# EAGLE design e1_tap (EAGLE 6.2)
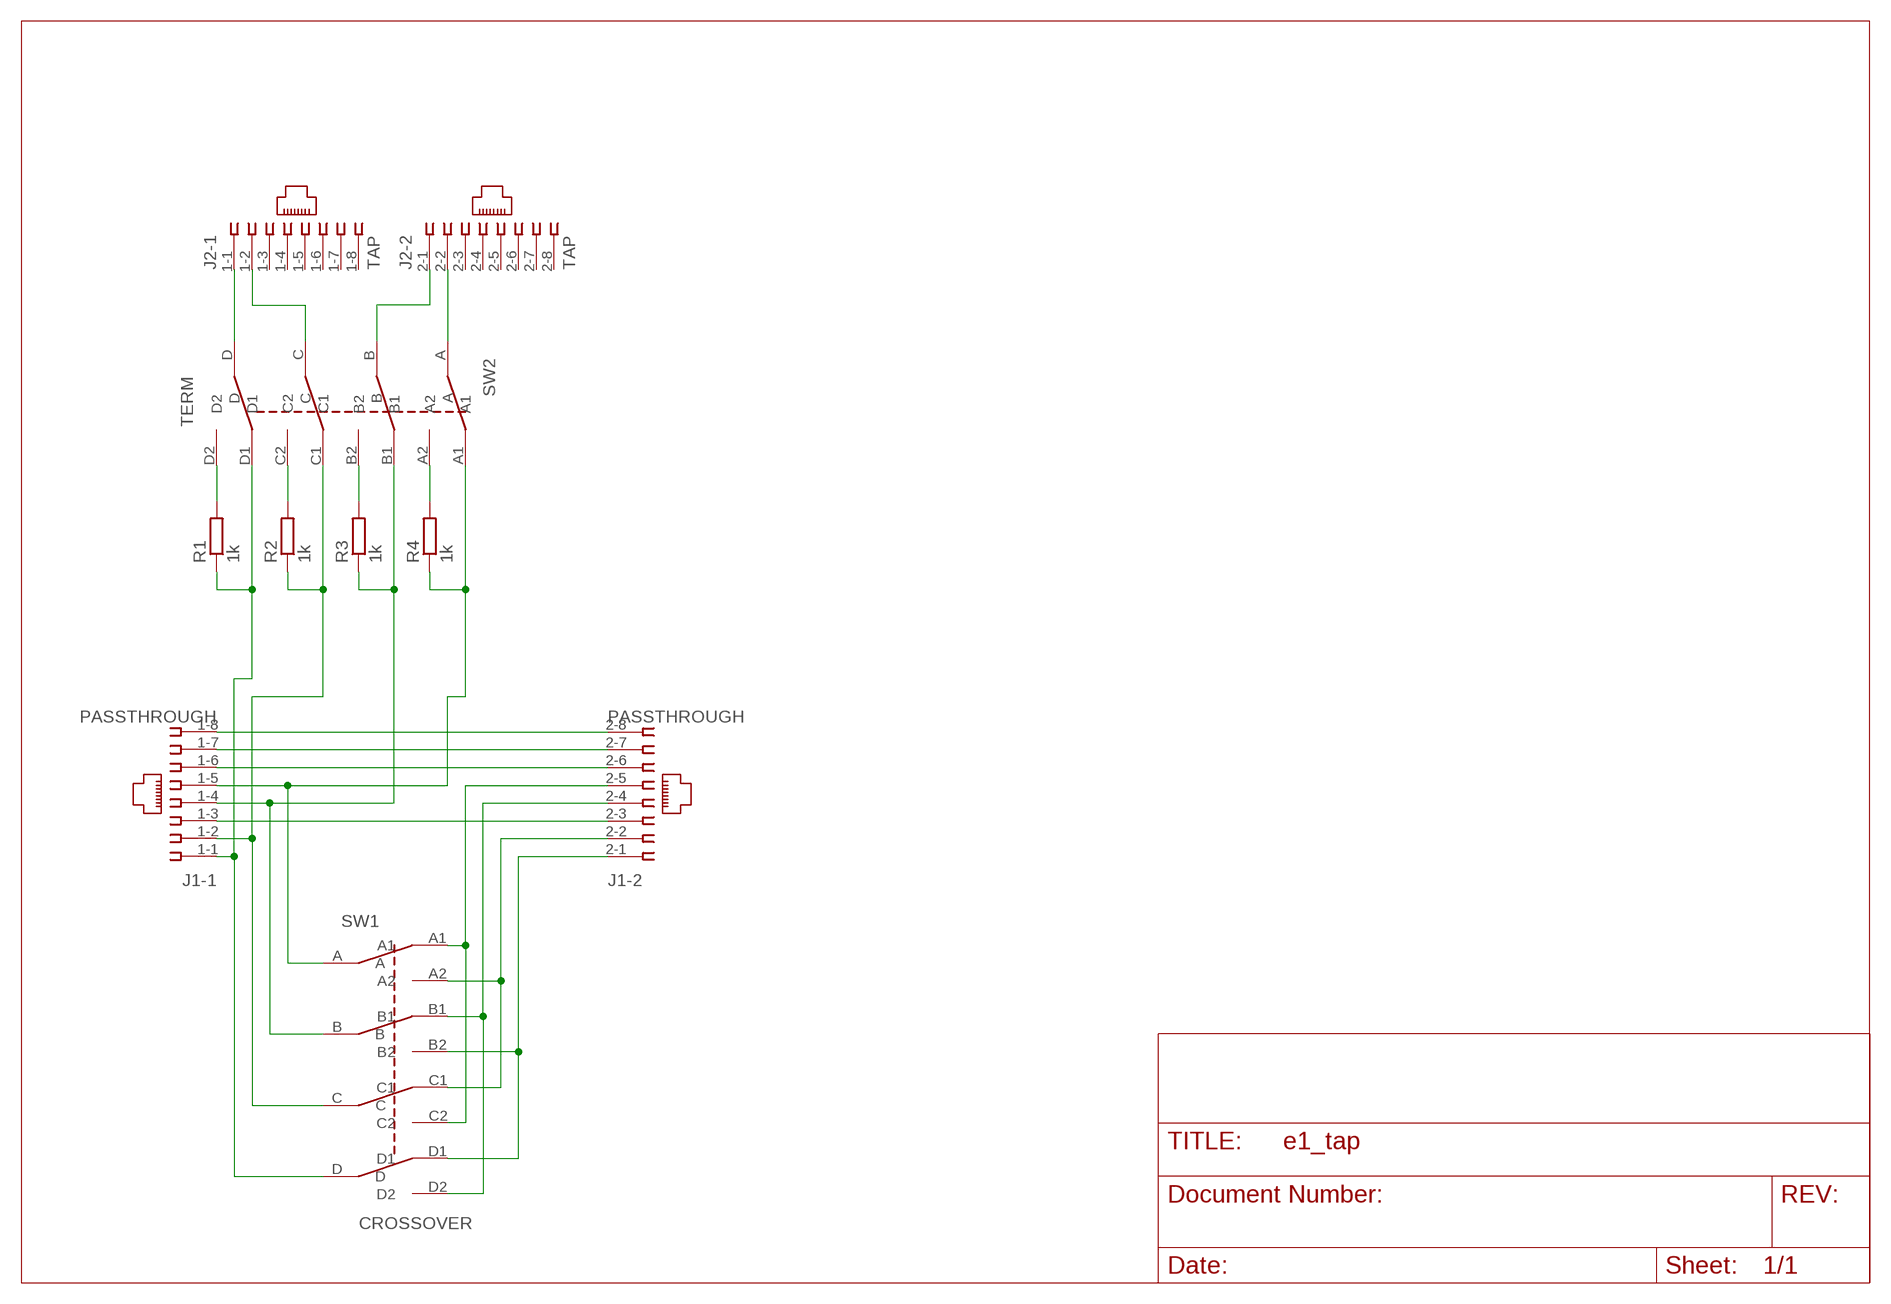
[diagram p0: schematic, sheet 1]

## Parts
J1  PASSTHROUGH  557560-1  [557560-1]
J2  TAP  557560-1  [557560-1]
R1  1k  R-EU_R0603  [R0603]
R2  1k  R-EU_R0603  [R0603]
R3  1k  R-EU_R0603  [R0603]
R4  1k  R-EU_R0603  [R0603]
SW1  CROSSOVER  SWITCH_4PDT  [4PDT_DIL12]
SW2  TERM  SWITCH_4PDT  [4PDT_DIL12]

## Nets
CROSS: J1.2-4 SW1.B1 SW1.D2
N$1: J1.1-8 J1.2-8
N$2: J1.1-7 J1.2-7
N$3: J1.1-6 J1.2-6
N$4: J1.1-3 J1.2-3
N$5: J1.1-2 R2.1 SW1.C SW2.C1
N$6: J1.1-1 R1.1 SW1.D SW2.D1
N$7: J1.1-4 R3.1 SW1.B SW2.B1
N$8: J1.1-5 R4.1 SW1.A SW2.A1
N$9: J1.2-5 SW1.A1 SW1.C2
N$10: J2.1-1 SW2.D
N$11: J1.2-2 SW1.A2 SW1.C1
N$12: J1.2-1 SW1.B2 SW1.D1
N$13: J2.1-2 SW2.C
N$14: J2.2-1 SW2.B
N$15: J2.2-2 SW2.A
N$16: R1.2 SW2.D2
N$17: R2.2 SW2.C2
N$18: R3.2 SW2.B2
N$19: R4.2 SW2.A2
Unconnected: J2.1-3 J2.1-4 J2.1-5 J2.1-6 J2.1-7 J2.1-8 J2.2-3 J2.2-4 J2.2-5 J2.2-6 J2.2-7 J2.2-8

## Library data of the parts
J1 J2 = con-amp:557560-1: AMP connector
R1-R4 = rcl:R-EU_: RESISTOR, European symbol
SW1 SW2 = laforge:SWITCH_4PDT

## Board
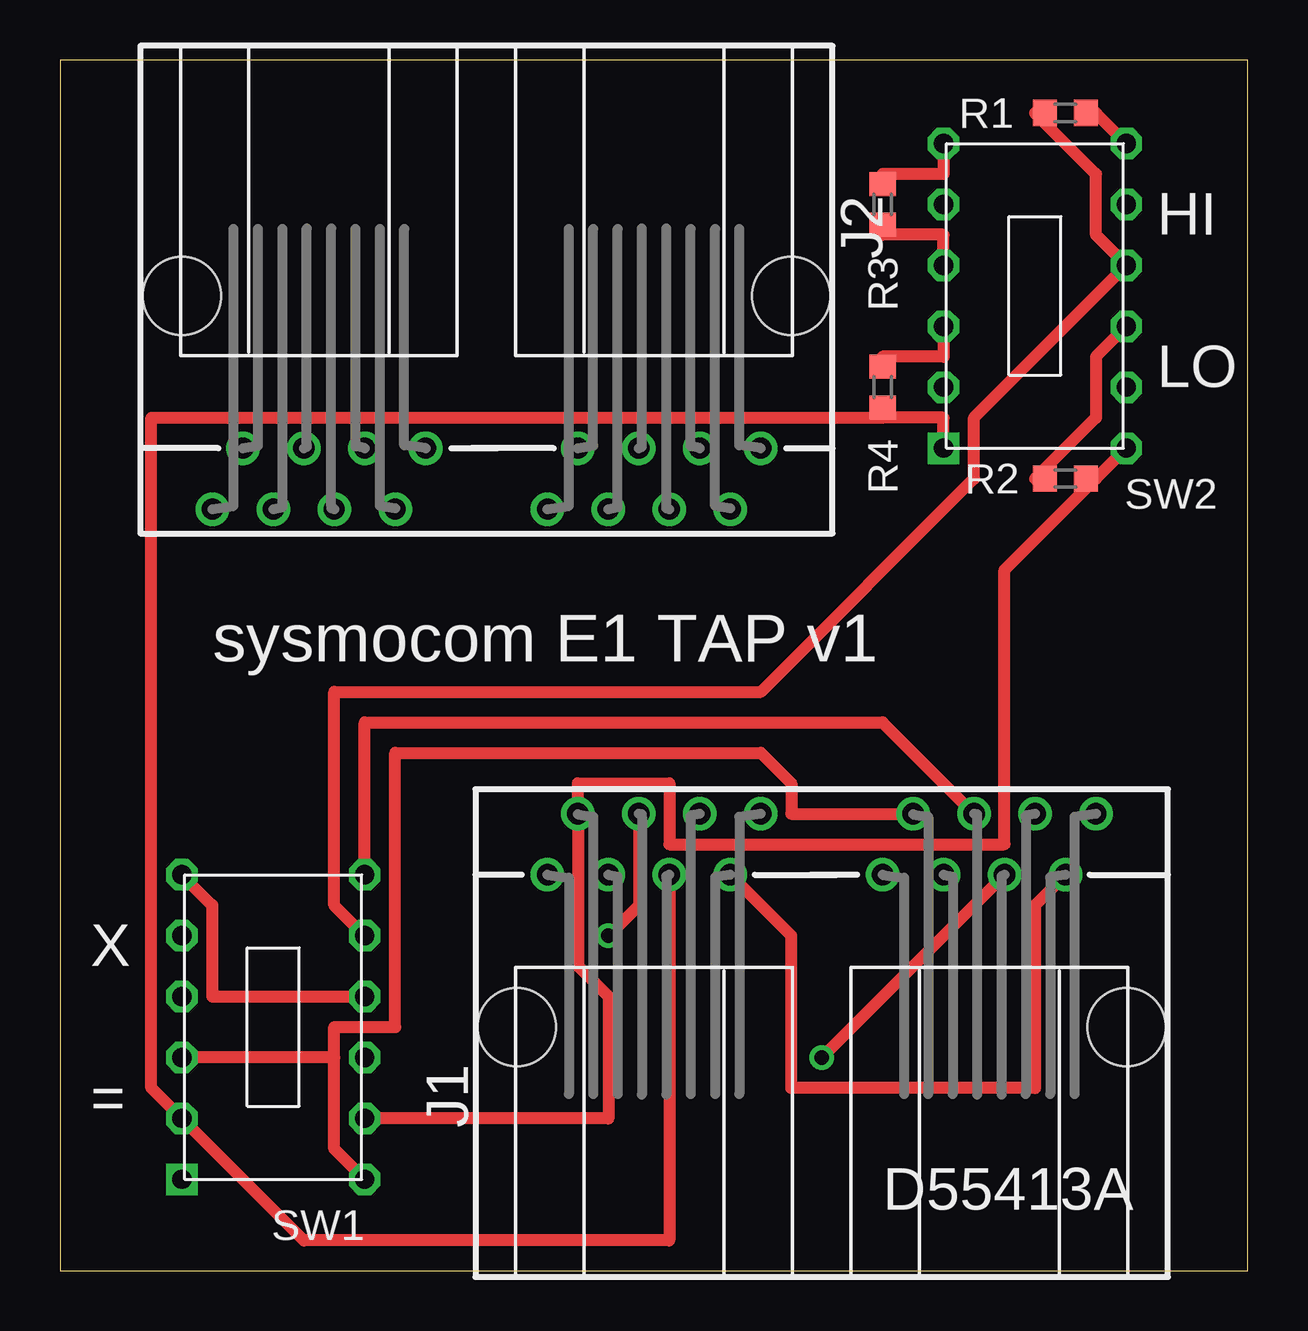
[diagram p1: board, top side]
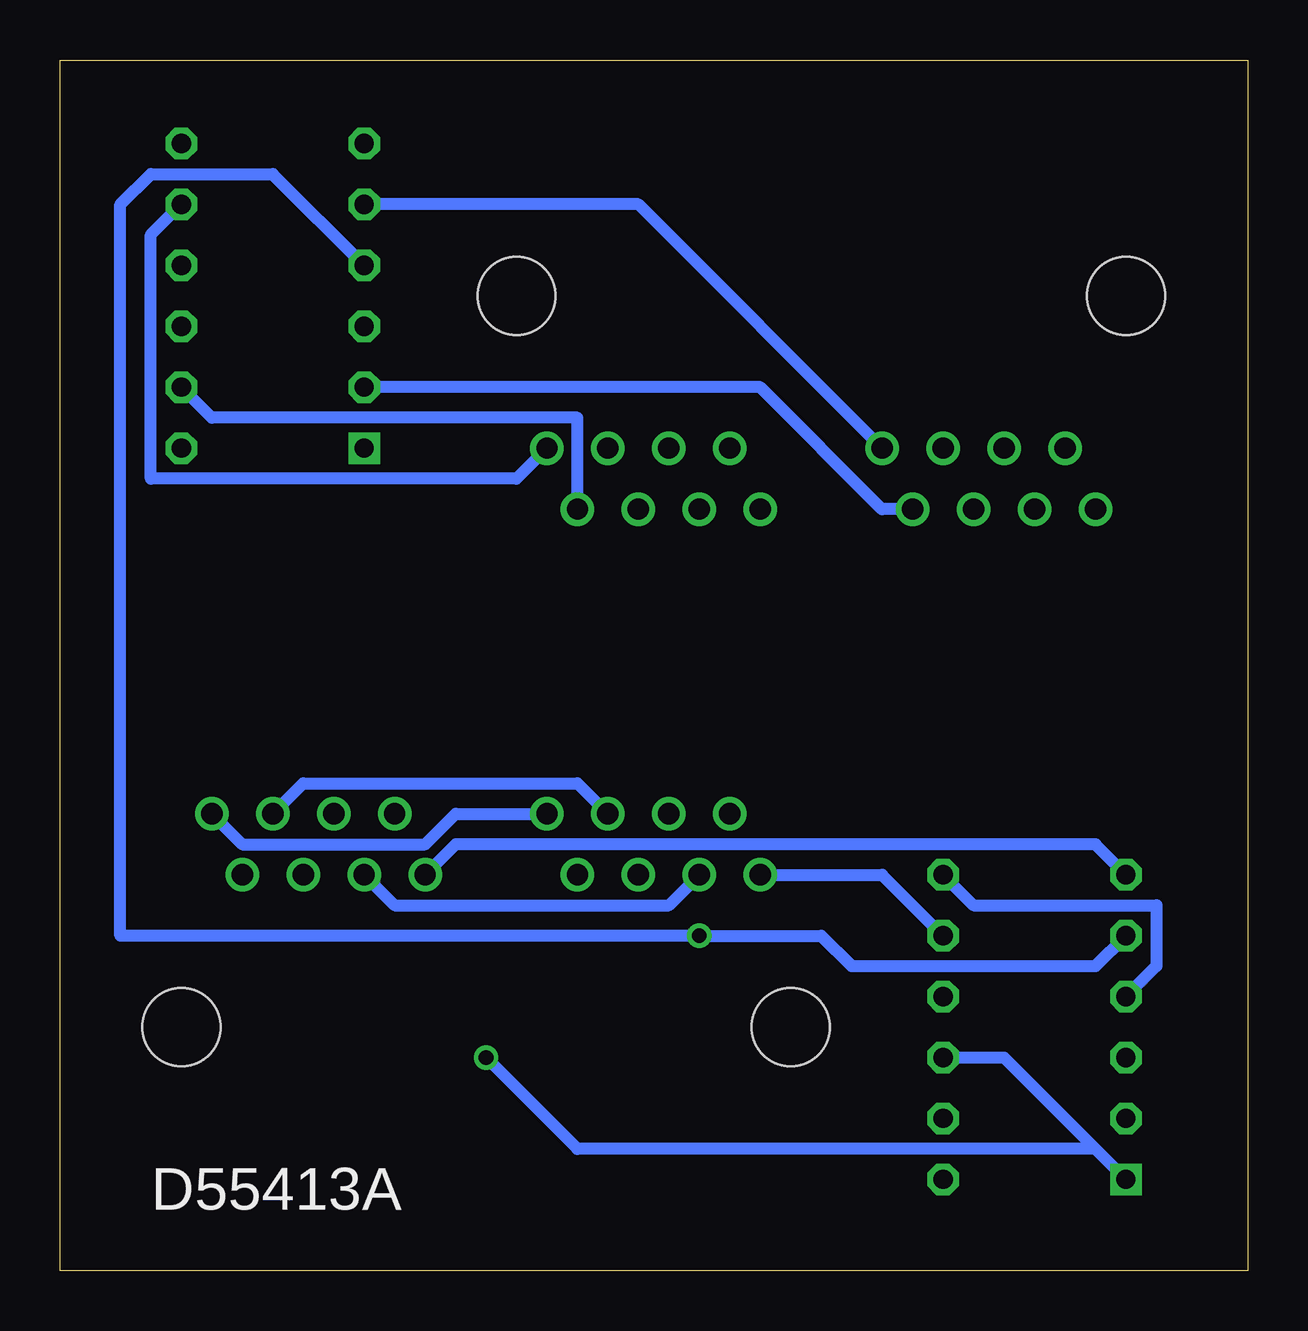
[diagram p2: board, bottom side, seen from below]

Size 49.51 x 50.47 mm. Coordinates in mm from the lower left corner, seen from the top.
Outline: 0,0 49.51,0 49.51,50.47 0,50.47 0,0
Copper layers (1*16): Top 0.035mm / dielectric 1.5mm / Bottom 0.035mm
Design rules: minimum track width 20mil, minimum drill 24mil, track to track 8mil, track to pad 8mil, pad to pad 8mil, via to via 8mil, smd to smd 8mil, copper to edge 40mil, drill to drill 8mil, minimum pad ring 10mil, minimum via ring 8mil, stop-mask expansion 4mil, vias tented up to drill 0mil, thermal gap 10mil

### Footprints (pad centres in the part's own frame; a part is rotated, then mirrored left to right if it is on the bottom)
557560-1 = drill 0.889: 1-1 -11.43,6.35; 1-2 -10.16,8.89; 1-3 -8.89,6.35; 1-4 -7.62,8.89; 1-5 -6.35,6.35; 1-6 -5.08,8.89; 1-7 -3.81,6.35; 1-8 -2.54,8.89; 2-1 2.54,6.35; 2-2 3.81,8.89; 2-3 5.08,6.35; 2-4 6.35,8.89; 2-5 7.62,6.35; 2-6 8.89,8.89; 2-7 10.16,6.35; 2-8 11.43,8.89 | hole 3.251: -12.7,0; 12.7,0
R0603 = smd 1 x 1.1: 1 -0.85,0; 2 0.85,0
4PDT_DIL12 = drill 0.8 octagon: A -3.81,3.81; A2 -1.27,3.81; B 3.81,3.81; B1 1.27,3.81; B2 6.35,3.81; C -3.81,-3.81; C1 -6.35,-3.81; C2 -1.27,-3.81; D 3.81,-3.81; D1 1.27,-3.81; D2 6.35,-3.81 | drill 0.8 square: A1 -6.35,3.81

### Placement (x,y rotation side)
J1  31.75,10.16 0 top
J2  17.78,40.64 180 top
R1  41.91,48.26 0 top
R2  41.91,33.02 180 top
R3  34.29,44.45 90 top
R4  34.29,36.83 90 top
SW1  8.89,10.16 90 top
SW2  40.64,40.64 90 top

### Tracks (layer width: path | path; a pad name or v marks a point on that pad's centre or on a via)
CROSS
  Top 0.508: J1.2-4 34.29,22.86 12.7,22.86 SW1.D2
  Bottom 0.508: SW1.B1 3.81,12.7 3.81,15.24 11.43,15.24 SW1.D2
N$1
  Bottom 0.508: J1.1-8 33.02,19.05 34.29,17.78 41.91,17.78 J1.2-8
N$2
  Top 0.508: J1.1-7 30.48,13.97 30.48,7.62 40.64,7.62 40.64,15.24 J1.2-7
N$3
  Bottom 0.508: J1.1-6 27.94,20.32 39.37,20.32 J1.2-6
N$4
  Bottom 0.508: J1.1-3 24.13,15.24 35.56,15.24 J1.2-3
N$5
  Top 0.508: SW2.C1 43.18,33.02 | SW1.C 22.86,6.35 22.86,11.43 21.59,12.7 J1.1-2 21.59,20.32 25.4,20.32 25.4,17.78 39.37,17.78 39.37,29.21 43.18,33.02 | 43.18,33.02 R2.1
N$6
  Top 0.508: R1.1 40.64,48.26 43.18,45.72 43.18,43.18 SW2.D1 38.1,35.56 38.1,33.02 29.21,24.13 11.43,24.13 11.43,15.24 SW1.D
  Bottom 0.508: SW1.D 15.24,16.51 J1.1-1
N$7  (via drill 0.61)
  Top 0.508: SW2.B1 36.83,43.18 34.29,43.18 R3.1 | v22.86,13.97 24.13,15.24 J1.1-4
  Bottom 0.508: SW1.B 6.35,12.7 16.51,12.7 17.78,13.97 v22.86,13.97 46.99,13.97 46.99,44.45 45.72,45.72 40.64,45.72 SW2.B1
N$8
  Top 0.508: 34.29,35.56 36.83,35.56 SW2.A1 | J1.1-5 25.4,1.27 10.16,1.27 SW1.A 3.81,7.62 3.81,35.56 34.29,35.56 | 34.29,35.56 R4.1
N$9  (via drill 0.61)
  Top 0.508: v31.75,8.89 J1.2-5
  Bottom 0.508: 6.35,5.08 10.16,8.89 SW1.C2 | 6.35,5.08 SW1.A1 | v31.75,8.89 27.94,5.08 6.35,5.08
N$10
  Bottom 0.508: SW2.D 45.72,43.18 45.72,33.02 30.48,33.02 J2.1-1
N$11
  Top 0.508: 11.43,8.89 SW1.A2 | 11.43,8.89 11.43,5.08 SW1.C1 | J1.2-2 30.48,19.05 30.48,20.32 29.21,21.59 13.97,21.59 13.97,10.16 11.43,10.16 11.43,8.89
N$12
  Top 0.508: SW1.D1 6.35,11.43 6.35,15.24 SW1.B2
  Bottom 0.508: J1.2-1 33.02,17.78 6.35,17.78 SW1.B2
N$13
  Bottom 0.508: SW2.C 43.18,35.56 27.94,35.56 J2.1-2
N$14
  Bottom 0.508: SW2.B 25.4,44.45 J2.2-1
N$15
  Bottom 0.508: SW2.A 20.32,36.83 15.24,31.75 J2.2-2
N$16
  Top 0.508: SW2.D2 43.18,48.26 R1.2
N$17
  Top 0.508: SW2.C2 43.18,38.1 43.18,35.56 40.64,33.02 R2.2
N$18
  Top 0.508: SW2.B2 36.83,45.72 34.29,45.72 R3.2
N$19
  Top 0.508: SW2.A2 36.83,38.1 34.29,38.1 R4.2

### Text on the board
tNames: HI | LO | sysmocom E1 TAP v1 | X | = | D55413A
bNames: D55413A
